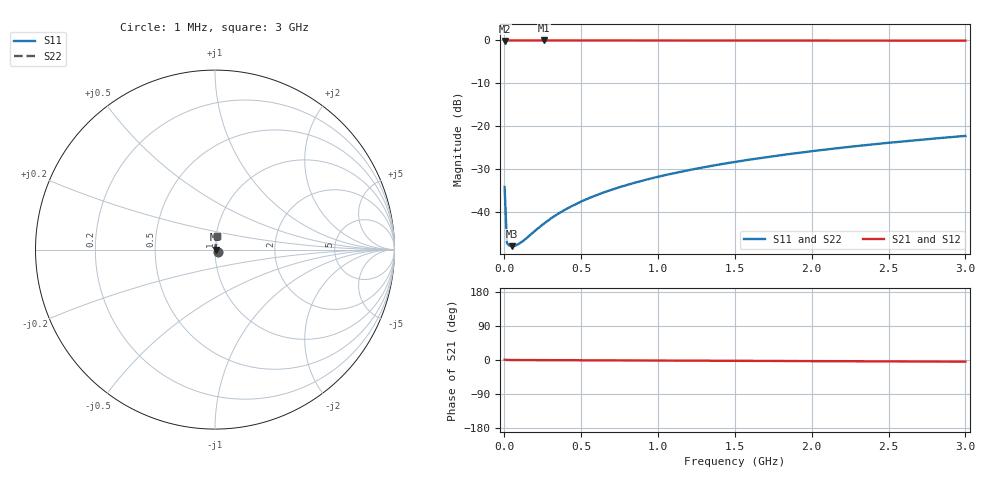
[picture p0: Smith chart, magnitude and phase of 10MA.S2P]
!Keysight Technologies,E4991B,MY54301043,A.02.04
!Date: Thu Nov 16 21:14:52 2023
!Data:
!Freq	S11	S21	S12	S22
# Hz S MA R 50
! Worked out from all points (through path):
!   201 points, 1 MHz to 3 GHz, reference 50 ohm
!   highest |S21| = -0.03 dB at 255.9 MHz (marker M1); lowest = -0.1 dB at 1 MHz (marker M2)
!   lowest |S11| = -48.0 dB at 45.98 MHz (marker M3), VSWR 1.01, Z = 50.4 + j0.0453 ohm
!   |S11| at or under -10 dB: start of sweep to end of sweep
!   |S22| runs from -48.0 to -22.3 dB; largest |S21 - S12| = 0
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1000000  0.01955 -44.6  0.9862 0.8  0.9862 0.8  0.01955 -44.6
1.5995e7  0.004338 -14.0  0.9958 0.1  0.9958 0.1  0.004338 -14.0
3.099e7  0.004059 -1.8  0.9959 0.0  0.9959 0.0  0.004059 -1.8
4.5985e7  0.00399 6.5  0.996 -0.0  0.996 -0.0  0.00399 6.5
7.5975e7  0.004094 19.9  0.9962 -0.1  0.9962 -0.1  0.004094 19.9
1.2096e8  0.004577 35.2  0.9963 -0.2  0.9963 -0.2  0.004577 35.2
1.95935e8  0.005969 51.8  0.9963 -0.3  0.9963 -0.3  0.005969 51.8
2.55915e8  0.007286 59.7  0.9963 -0.4  0.9963 -0.4  0.007286 59.7
3.15895e8  0.008714 64.7  0.9963 -0.5  0.9963 -0.5  0.008714 64.7
3.6088e8  0.009801 67.5  0.9963 -0.5  0.9963 -0.5  0.009801 67.5
4.2086e8  0.01127 70.1  0.9962 -0.6  0.9962 -0.6  0.01127 70.1
5.1083e8  0.01351 73.0  0.9961 -0.7  0.9961 -0.7  0.01351 73.0
6.15795e8  0.01612 75.2  0.996 -0.9  0.996 -0.9  0.01612 75.2
7.5075e8  0.01948 77.1  0.9958 -1.1  0.9958 -1.1  0.01948 77.1
8.85705e8  0.02286 78.3  0.9956 -1.3  0.9956 -1.3  0.02286 78.3
1.005665e9  0.02585 79.1  0.9954 -1.5  0.9954 -1.5  0.02585 79.1
1.245585e9  0.03187 80.1  0.995 -1.8  0.995 -1.8  0.03187 80.1
1.5005e9  0.0383 80.8  0.9946 -2.2  0.9946 -2.2  0.0383 80.8
1.725425e9  0.04402 81.2  0.9942 -2.5  0.9942 -2.5  0.04402 81.2
2.01033e9  0.0513 81.4  0.9936 -2.9  0.9936 -2.9  0.0513 81.4
2.505165e9  0.06406 81.4  0.9924 -3.7  0.9924 -3.7  0.06406 81.4
3e9  0.07693 81.2  0.9911 -4.4  0.9911 -4.4  0.07693 81.2
